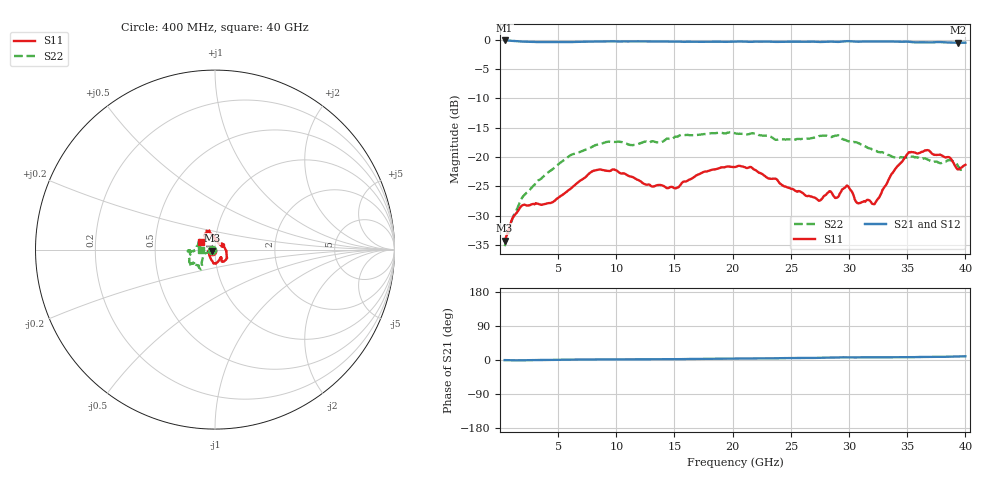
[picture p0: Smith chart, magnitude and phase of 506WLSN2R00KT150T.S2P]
!  American Technical Ceramics  Date:  8/31/2012
!  One Norden Lane
!  Huntington Station,  NY.  11746-2102
!  Tel:  (631) 622-4700  Fax:  (631) 622-4748
!  Part Number  506WLSN2R00KG150T
!  Description:  Ultra-Broadband Inductor
!  Application:  Ultra-broadband DC block decoupling, bias tee
# GHZ S DB R 50
! Freq  |S11|  S11 Ph  |S21|  S21 Ph  |S12|  S12 Ph  |S22|  S22 Ph
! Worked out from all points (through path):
!   401 points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, 400 MHz to 40 GHz, reference 50 ohm
!   highest |S21| = -0.14 dB at 400 MHz (marker M1); lowest = -0.5 dB at 39.41 GHz (marker M2)
!   lowest |S11| = -34.2 dB at 400 MHz (marker M3), VSWR 1.04, Z = 48.2 - j0.508 ohm
!   |S11| at or under -10 dB: start of sweep to end of sweep
!   |S22| runs from -35.2 to -15.8 dB; largest |S21 - S12| = 0.005
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0.4  -34.24 -164.2  -0.14 -0.3  -0.13 -0.3  -35.20 -163.3
1.192  -30.08 -157.3  -0.23 -0.8  -0.23 -0.9  -29.89 -153.0
2.083  -28.12 -164.3  -0.35 -0.7  -0.34 -0.7  -26.49 -158.5
4.459  -27.76 -144.5  -0.41 0.4  -0.42 0.3  -22.18 -148.4
7.033  -23.88 -105.9  -0.36 1.3  -0.37 1.3  -19.00 -130.3
8.122  -22.31 -97.1  -0.32 1.4  -0.33 1.3  -18.06 -124.8
9.805  -22.13 -85.8  -0.29 1.4  -0.30 1.4  -17.43 -127.7
13.666  -24.77 -54.3  -0.32 1.9  -0.33 1.9  -17.55 -148.1
15.151  -25.31 -53.5  -0.33 2.2  -0.34 2.3  -16.55 -149.4
17.428  -22.61 -60.2  -0.36 3.0  -0.37 3.0  -16.14 -146.9
20.2  -21.72 -46.9  -0.34 4.0  -0.35 4.1  -15.94 -148.8
21.685  -21.87 -34.3  -0.37 4.3  -0.37 4.4  -15.95 -153.5
26.833  -26.79 36.6  -0.34 5.4  -0.34 5.5  -16.75 -177.1
28.912  -26.96 36.5  -0.38 6.6  -0.38 6.6  -16.37 -175.8
29.803  -24.86 30.1  -0.26 7.0  -0.26 7.0  -17.19 -176.8
30.694  -27.83 25.9  -0.35 6.9  -0.35 7.0  -17.56 -175.8
32.08  -28.02 54.3  -0.32 7.1  -0.32 7.2  -18.80 -177.0
33.466  -23.62 92.2  -0.32 7.2  -0.30 7.4  -19.68 171.1
35.347  -19.14 106.4  -0.41 7.2  -0.40 7.3  -19.94 149.0
38.515  -20.01 127.4  -0.49 8.6  -0.48 8.7  -20.56 168.3
39.406  -22.12 140.7  -0.53 9.3  -0.51 9.6  -21.73 170.8
40  -21.33 151.4  -0.52 9.8  -0.51 9.9  -22.17 179.9
